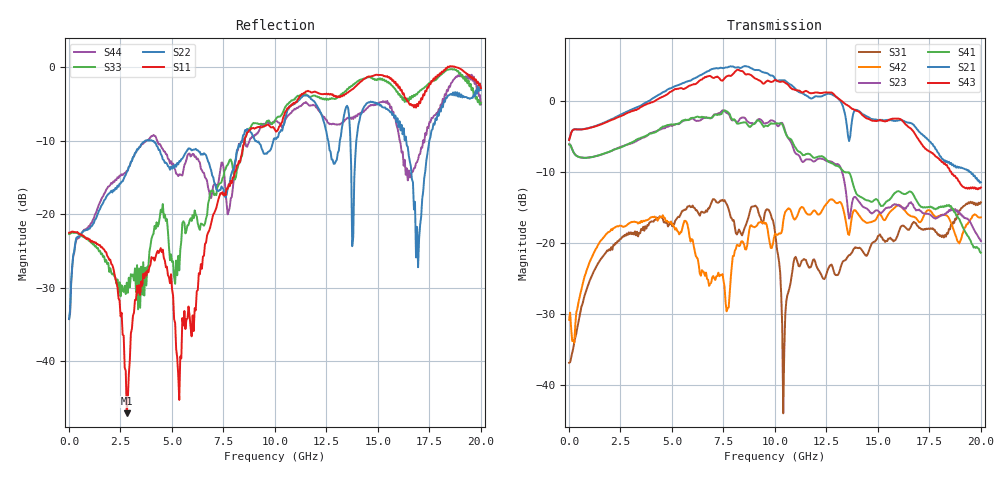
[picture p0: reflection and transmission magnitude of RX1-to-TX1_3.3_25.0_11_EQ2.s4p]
!Agilent Technologies,N5225A,MY51451112,A.09.50.13
!Agilent N5225A: A.09.50.13
!Date: Wednesday, January 31, 2018 11:02:59
!Correction: S11(Full 4 Port(1,2,3,4))
!S12(Full 4 Port(1,2,3,4))
!S13(Full 4 Port(1,2,3,4))
!S14(Full 4 Port(1,2,3,4))
!S21(Full 4 Port(1,2,3,4))
!S22(Full 4 Port(1,2,3,4))
!S23(Full 4 Port(1,2,3,4))
!S24(Full 4 Port(1,2,3,4))
!S31(Full 4 Port(1,2,3,4))
!S32(Full 4 Port(1,2,3,4))
!S33(Full 4 Port(1,2,3,4))
!S34(Full 4 Port(1,2,3,4))
!S41(Full 4 Port(1,2,3,4))
!S42(Full 4 Port(1,2,3,4))
!S43(Full 4 Port(1,2,3,4))
!S44(Full 4 Port(1,2,3,4))
!S4P File: Measurements: <S11,S12,S13,S14>,
!<S21,S22,S23,S24>,
!<S31,S32,S33,S34>,
!<S41,S42,S43,S44>:
# Hz S  RI  R 50
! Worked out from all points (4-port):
!   401 points, 10 MHz to 20 GHz, reference 50 ohm
!   strongest paths, dB at 10 MHz, 5.008 GHz, 10.01 GHz, 15 GHz, 20 GHz:
!     S43: -5.5, 1.5, 3.0, -2.7, -12.2
!     S21: -5.4, 2.0, 3.2, -2.6, -11.4
!     S41: -6.1, -3.3, -3.1, -14.0, -21.4
!     S23: -6.1, -3.5, -2.9, -15.4, -19.7
!     S42: -30.8, -17.3, -18.7, -16.1, -16.4
!     S31: -36.9, -17.6, -18.4, -19.0, -14.2
!   lowest |S11| = -47.1 dB at 2.809 GHz (marker M1), VSWR 1.01, Z = 49.7 - j0.333 ohm
!   |S11| at or under -10 dB: start of sweep to 8.529 GHz
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1e7  -0.0747 -0.00312  -0.000208 0.000458  0.0136 0.000711  -0.000103 0.000482
     0.5362 0.00727  -0.0135 0.0139  -0.498 0.00459  0.0265 0.0118
     0.0143 0.00085  5.21e-05 0.000525  -0.0732 -0.00405  0.000172 0.000743
     -0.4974 0.00473  0.0262 0.0117  0.5338 0.00636  -0.0129 0.0145
2.8086e9  -0.00291 -0.00335  0.0165 0.00256  0.0549 0.1042  0.018 0.000224
          0.5635 -0.6298  0.1935 0.00295  -0.2418 0.4321  0.0999 0.0919
          0.0564 0.1023  0.0198 0.00315  0.0193 0.0283  0.0215 0.000296
          -0.1797 0.4609  0.0936 0.0949  0.4053 -0.7193  0.1903 -0.0506
7.156425e9  -0.0143 0.1094  0.0157 -0.0199  0.1288 0.0965  0.00144 -0.0336
            -1.717 0.0217  0.1269 -0.0745  0.7796 -0.2237  0.0534 0.0169
            0.158 0.1136  0.0246 -0.0277  0.0254 0.1323  0.00921 -0.049
            0.6138 -0.5308  0.0583 -0.00138  -1.297 0.7256  0.1099 -0.1119
8.8056e9  0.00708 0.3738  0.012 -0.0143  0.1243 0.1063  -0.00647 -0.0152
          -0.6333 1.607  -0.0971 0.348  0.1436 -0.6891  0.0192 0.1306
          0.1305 0.1107  0.00148 -0.0236  0.0577 0.3791  -0.0138 -0.0257
          -0.1624 -0.6412  0.00243 0.1324  0.2817 1.517  0.263 0.194
1.090455e10  0.2032 0.5336  -0.0114 -0.0337  0.0376 0.0392  -0.0304 0.00991
             1.059 0.6968  0.4063 0.3817  -0.4466 -0.1206  0.1034 0.1589
             0.0339 0.0648  -0.0189 -0.00956  0.242 0.5484  -0.0447 0.00385
             -0.4826 0.1219  0.094 0.1163  1.22 -0.0171  0.4479 -0.2366
1.570215e10  0.5865 0.5498  -0.0271 -0.00512  -0.0478 0.1035  -0.0203 0.0227
             -0.2381 -0.6983  0.274 0.3828  -0.0626 0.1735  0.1207 0.1044
             -0.0414 0.0973  -0.0217 0.00137  0.6429 0.3751  -0.016 0.0286
             0.1187 0.1793  0.1266 0.1162  -0.7508 -0.0813  0.0955 -0.4776
2e10  0.7146 0.0583  0.023 0.035  -0.0801 0.1706  0.0345 0.0208
      -0.0723 0.2585  0.6931 0.0769  0.1017 -0.019  0.1504 0.0438
      -0.0838 0.1752  0.00635 0.0478  0.5687 -0.0319  0.0478 0.0206
      0.0125 -0.0845  0.1449 0.0454  0.1946 0.1516  -0.153 -0.5346
